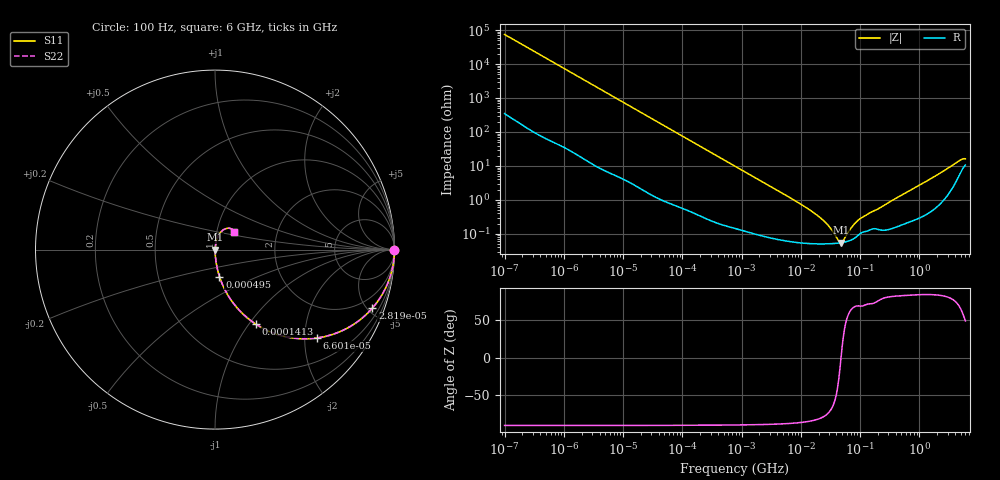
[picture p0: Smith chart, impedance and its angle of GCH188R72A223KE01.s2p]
!Murata Part Number: GCH188R72A223KE01
!These Parameters are Measured in Series Mode Connection
!Data Generated on Mar 13, 2026
!  o--ll--o
!Port1  Port2
!  o------o
!Operation Temp=25[degC], DC Bias Voltage=0[V]
!Freq. Start=100[Hz] Stop=6[GHz] 401[Steps]
# Hz S RI R 50
!Freq.(Hz) S11(Real) S11(Imag) S21(Real) S21(Imag) S12(Real) S12(Imag) S22(Real) S22(Imag)
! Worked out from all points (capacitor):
!   401 points, 100 Hz to 6 GHz, reference 50 ohm
!   read as one part in series: C = 21.4 nF near 109 Hz
!   lowest |Z| = 55 mohm at 47.65 MHz (marker M1)
!   series resonance near 47.72 MHz, so ESL is about 520 pH
!   S11 on the Smith chart (normalised r, x): 100 Hz: open; 28.19 kHz: 1.03, -5.37; 66 kHz: 1.01, -2.30; 141.3 kHz: 1.01, -1.08; 495 kHz: 1.00, -0.31; 6 GHz: 1.21, +0.25
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100  1 -0.00134  8.1e-06 0.00134  8.1e-06 0.00134  1 -0.00134
2008  0.9992 -0.0267  0.000841 0.0267  0.000841 0.0267  0.9992 -0.0267
8801  0.9859 -0.1151  0.0141 0.1151  0.0141 0.1151  0.9859 -0.1151
28191  0.8767 -0.3261  0.1233 0.3261  0.1233 0.3261  0.8767 -0.3261
40335  0.7776 -0.413  0.2224 0.413  0.2224 0.413  0.7776 -0.413
66005  0.5684 -0.492  0.4316 0.492  0.4316 0.492  0.5684 -0.492
141303  0.2266 -0.4146  0.7734 0.4146  0.7734 0.4146  0.2266 -0.4146
241822  0.0926 -0.2854  0.9074 0.2854  0.9074 0.2854  0.0926 -0.2854
495019  0.025 -0.1504  0.975 0.1504  0.975 0.1504  0.025 -0.1504
774597  0.0111 -0.0978  0.9889 0.0978  0.9889 0.0978  0.0111 -0.0978
2481164  0.00179 -0.031  0.9982 0.031  0.9982 0.031  0.00179 -0.031
1.555665e7  0.000534 -0.0045  0.9995 0.0045  0.9995 0.0045  0.000534 -0.0045
2.662322e7  0.000513 -0.00203  0.9995 0.00203  0.9995 0.00203  0.000513 -0.00203
4.35672e7  0.000538 -0.000301  0.9995 0.000301  0.9995 0.000301  0.000538 -0.000301
4.764863e7  0.00055 -4.6e-06  0.9995 4.6e-06  0.9995 4.6e-06  0.00055 -4.6e-06
5.211241e7  0.000565 0.000293  0.9994 -0.000293  0.9994 -0.000293  0.000565 0.000293
7.129496e7  0.000668 0.00138  0.9993 -0.00138  0.9993 -0.00138  0.000668 0.00138
9.326766e7  0.00092 0.00237  0.9991 -0.00237  0.9991 -0.00237  0.00092 0.00237
3.124326e8  0.00143 0.00851  0.9986 -0.00851  0.9986 -0.00851  0.00143 0.00851
2.34314e9  0.0121 0.0626  0.9879 -0.0626  0.9879 -0.0626  0.0121 0.0626
4.586474e9  0.0598 0.1167  0.9402 -0.1167  0.9402 -0.1167  0.0598 0.1167
6e9  0.1075 0.0994  0.8925 -0.0994  0.8925 -0.0994  0.1075 0.0994
